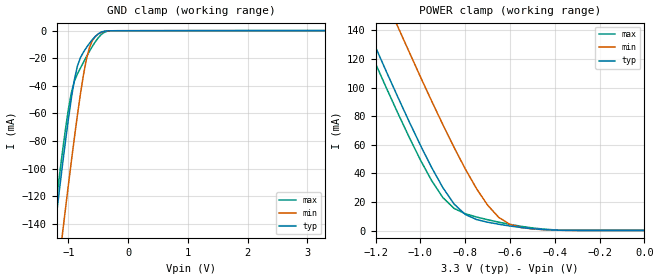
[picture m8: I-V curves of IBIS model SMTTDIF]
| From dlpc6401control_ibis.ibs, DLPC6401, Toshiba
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[Model]   SMTTDIF
Model_type   Input
Polarity   Non-Inverting
Vinl =   0.8000V
Vinh =   2.0000V
C_comp   1.443pF   NA   NA
|Variable   typ   min   max
[Voltage range]  3.3   3.0   3.6
[Temperature Range]   25.0000   125.000   0.000
[POWER Clamp Reference]   3.3000V   3.0000V   3.6000V
[GND Clamp Reference]   0.000V   0.000V   0.000V
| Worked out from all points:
|   GND clamp passes 1 mA (typ) near -0.45 V on its own axis
|   POWER clamp passes 1 mA (typ) near -0.48 V on its own axis
[GND_clamp]
| voltage   I(typ)   I(min)   I(max)
-3.3V     -944.9mA   -993.6mA   -933.7mA
-1.3V     -169.6mA   -220.5mA   -158.5mA
-1.25V    -151.2mA   -201.9mA   -140.2mA
-1.2V     -132.9mA   -183.4mA   -122.2mA
-1.1V     -97.21mA   -147mA     -87.48mA
-1V       -63.64mA   -111.4mA   -56.63mA
-900mV    -35.31mA   -77.27mA   -36.42mA
-800mV    -19.56mA   -45.93mA   -27.09mA
-700mV    -12.24mA   -20.73mA   -18.9mA
-600mV    -6.457mA   -7.167mA   -11.32mA
-450mV    -981uA     -1.198mA   -2.726mA
3.3V      72.06uA    62.27uA    111.7uA
[POWER_clamp]
| voltage   I(typ)   I(min)   I(max)
-3.3V     917.5mA    964.8mA    906.4mA
-1.3V     164.1mA    213.9mA    152.5mA
-1.25V    146.1mA    195.8mA    134.5mA
-1.2V     128.2mA    177.9mA    116.7mA
-1.1V     93.15mA    142.3mA    81.93mA
-950mV    44.17mA    90.68mA    34.98mA
-850mV    18.62mA    58.27mA    15.52mA
-750mV    7.719mA    29.47mA    9.484mA
-650mV    4.383mA    9.19mA     5.848mA
-600mV    3.161mA    4.286mA    4.295mA
-500mV    1.278mA    1.099mA    1.824mA
0V        72.06uA    38.01uA    111.9uA
